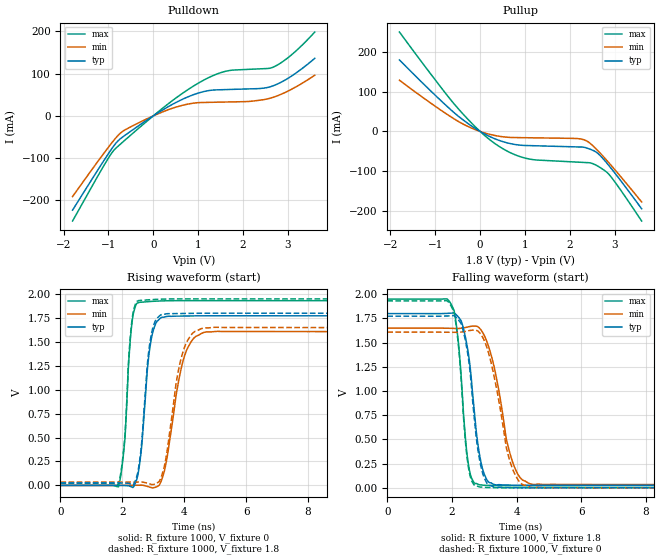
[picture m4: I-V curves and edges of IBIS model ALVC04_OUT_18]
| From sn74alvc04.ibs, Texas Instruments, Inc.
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[Model]   ALVC04_OUT_18
Model_type  Output
Vref =   0
Rref =   1000
Cref =   30p
Vmeas =   0.9
| variable   typ   min   max
C_comp   6.69pF   4.52pF   9.57pF
| C_pullup   6.68pF   5.77pF   7.77pF
| C_pulldown   6.70pF   4.52pF   9.57pF
[Temperature Range]   40   100   -40
| Ambient temperature   25   85   -40
[Voltage range]   1.8   1.65   1.95
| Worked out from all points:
|   slope of the pulldown table from 0 to 0.27 V, typ, clamps not added: 15.1 ohm
|   slope of the pullup table from 0 to 0.27 V, typ, clamps not added: 17.2 ohm
|   rising waveform, R_fixture 1000, V_fixture 0: 20-80 % time 273ps typ, 488ps min, 209ps max; typ from 0 V to 1.77 V
|   falling waveform, R_fixture 1000, V_fixture 1.8: 20-80 % time 355ps typ, 545ps min, 268ps max; typ from 1.8 V to 0.026 V
|   rising waveform, R_fixture 1000, V_fixture 1.8: 20-80 % time 266ps typ, 454ps min, 208ps max; typ from 0.026 V to 1.8 V
|   falling waveform, R_fixture 1000, V_fixture 0: 20-80 % time 349ps typ, 538ps min, 267ps max; typ from 1.77 V to 0 V
[Pulldown]
| ALVC04_OUT_18
|   Voltage   I(typ)   I(min)   I(max)
-1.8V     -222.9mA   -190.8mA   -248.7mA
-1.16V    -115.3mA   -96.71mA   -128.2mA
-900mV    -73.87mA   -60.44mA   -84.04mA
-650mV    -47.46mA   -34.43mA   -59.1mA
120mV     8.172mA    5.585mA    10.53mA
835mV     47.64mA    29.07mA    66.4mA
1.41V     61.46mA    32.32mA    98.6mA
1.715V    62.48mA    32.95mA    107.5mA
2.17V     63.88mA    34.47mA    110.2mA
2.72V     73.13mA    45.65mA    117.6mA
3.115V    96.46mA    64.78mA    147.4mA
3.6V      136.1mA    96.08mA    198.3mA
[Pullup]
| ALVC04_OUT_18
|   Voltage   I(typ)   I(min)   I(max)
-1.8V     180.1mA    129.1mA    250.4mA
-595mV    48.7mA     32.74mA    71.37mA
-165mV    11.71mA    7.199mA    18.08mA
220mV     -13.11mA   -7.415mA   -21.29mA
625mV     -29.35mA   -14.72mA   -50.81mA
1.03V     -35.42mA   -15.77mA   -67.83mA
2.14V     -38.87mA   -17.72mA   -77.04mA
2.35V     -40.8mA    -22.55mA   -78.25mA
2.605V    -53.56mA   -46.2mA    -86.16mA
2.855V    -83.9mA    -77.05mA   -106.1mA
3.1V      -119mA     -109.2mA   -142.4mA
3.6V      -194.7mA   -177.6mA   -225.5mA
[Ramp]
| ALVC04_OUT_18
| variable   typ   min   max
dV/dt_r   1.08/2.84E-10   0.98/5.07E-10   1.17/2.32E-10
dV/dt_f   1.07/3.72E-10   0.98/5.94E-10   1.16/2.79E-10
R_load = 1000
[Rising Waveform]
| ALVC04_OUT_18
R_fixture =   1000
C_fixture =   0
L_fixture =   0
V_fixture =   0
V_fixture_min = 0
V_fixture_max = 0
|   Time   V(typ)   V(min)   V(max)
0s        30.1pV     5.265nV    21.7pV
1.875ns   543uV      182.9uV    -15.67mV
2.08ns    -1.38mV    473.8uV    473.2mV
2.31ns    -17.22mV   1.122mV    1.696V
2.575ns   265.4mV    2.219mV    1.915V
2.85ns    1.341V     -14.03mV   1.922V
3.075ns   1.689V     -18.9mV    1.927V
4.015ns   1.771V     1.36V      1.932V
4.71ns    1.774V     1.605V     1.932V
40ns      1.773V     1.608V     1.932V
[Falling Waveform]
| ALVC04_OUT_18
R_fixture =   1000
C_fixture =   0
L_fixture =   0
V_fixture =   1.8
V_fixture_min = 1.65
V_fixture_max = 1.95
|   Time   V(typ)   V(min)   V(max)
0s        1.8V       1.65V      1.95V
2ns       1.805V     1.647V     1.88V
2.2ns     1.763V     1.646V     1.495V
2.405ns   1.574V     1.655V     557.1mV
2.51ns    1.379V     1.663V     237.4mV
2.87ns    309.6mV    1.642V     29.51mV
3.28ns    36.94mV    1.282V     22.94mV
3.87ns    26.5mV     270.8mV    21.43mV
4.495ns   24.63mV    34.22mV    21.52mV
40ns      25.59mV    33.88mV    21.73mV
[Rising Waveform]
| ALVC04_OUT_18
R_fixture =   1000
C_fixture =   0
L_fixture =   0
V_fixture =   1.8
V_fixture_min = 1.65
V_fixture_max = 1.95
|   Time   V(typ)   V(min)   V(max)
0s        25.59mV    33.88mV    21.73mV
1.875ns   26.02mV    34.04mV    6.315mV
2.08ns    24.09mV    34.25mV    503.6mV
2.3ns     10.12mV    34.68mV    1.696V
2.53ns    193mV      35.31mV    1.933V
2.93ns    1.567V     11.24mV    1.942V
3.435ns   1.795V     335.9mV    1.949V
3.96ns    1.798V     1.397V     1.951V
4.655ns   1.8V       1.647V     1.951V
40ns      1.8V       1.65V      1.95V
[Falling Waveform]
| ALVC04_OUT_18
R_fixture =   1000
C_fixture =   0
L_fixture =   0
V_fixture =   0
V_fixture_min = 0
V_fixture_max = 0
|   Time   V(typ)   V(min)   V(max)
0s        1.773V     1.608V     1.932V
1.995ns   1.778V     1.607V     1.864V
2.195ns   1.736V     1.606V     1.482V
2.395ns   1.552V     1.615V     561.7mV
2.505ns   1.345V     1.623V     218.8mV
2.87ns    259.7mV    1.595V     7.42mV
3.215ns   20.41mV    1.284V     1.522mV
3.83ns    1.05mV     235.4mV    -289.3uV
4.48ns    -924.5uV   286.5uV    -213uV
40ns      30.1pV     5.256nV    21.34pV
